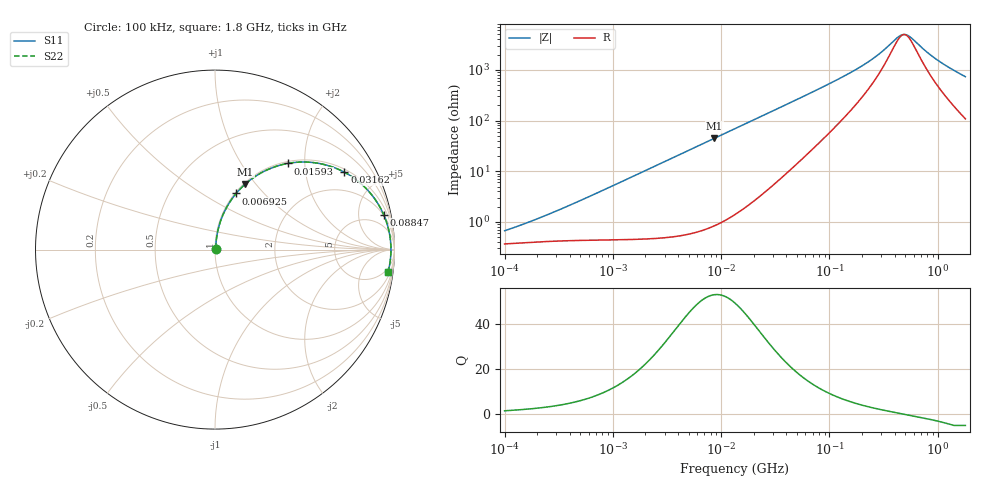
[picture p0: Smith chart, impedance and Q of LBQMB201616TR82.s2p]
! LBQMB201616TR82  S-PARAMETER MODEL  ( General Type )
! Model Generated by TAIYO YUDEN Corporation (http://www.ty-top.com)
! Version 1.0
! TAIYO YUDEN Control No. 191025NI43SB-FBB
! Copyright(c) 2019 TAIYO YUDEN CO.,LTD. All Rights Reserved.
! Product Description (link to TY-COMPAS)
! https://ds.yuden.co.jp/TYCOMPAS/or/detail?pn=LBQMB201616TR82J&u=M
! Products Name : Inductors
! Characteristics :
!  Inductance : 0.82 uH , SRF(min) : 250 MHz , DC Resistance(max) : 0.442 Ohm , Rated Current : 390 mA
!  Case Size : 2.0 x 1.6 / 0.079 x 0.063 [mm/inch] , Thickness : 1.6 / 0.063 [mm/inch]
!  (Conditions: Temperature = 25 degC , DC Bias Current/Voltage = 0A / 0V)
! External Node Assignments :
!  1  o---GGG---o  2
! GND o---------o GND
! Frequency Range : 0.1MHz  -  1800MHz  [ 402 STEP ]
# MHz S RI R 50
! Freq[MHz].  S11 Real  S11 Imag  S21 Real  S21 Imag  S12 Real  S12 Imag  S22 Real  S22 Imag
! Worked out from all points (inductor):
!   401 points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, 100 kHz to 1.8 GHz, reference 50 ohm
!   read as one part in series: L = 844 nH near 230 kHz
!   highest Q = 53.2 at 8.633 MHz (marker M1), where L = 820 nH
!   self-resonance near 489.8 MHz
!   S11 on the Smith chart (normalised r, x): 100 kHz: 1.01, +0.01; 6.925 MHz: 1.01, +0.71; 15.93 MHz: 1.04, +1.64; 31.62 MHz: 1.12, +3.27; 88.47 MHz: 1.89, +9.34; 1.8 GHz: 3, -15
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0.1  0.0037 0.00556  0.9963 -0.00556  0.9963 -0.00556  0.0037 0.00556
0.203473  0.00413 0.0109  0.9959 -0.0109  0.9959 -0.0109  0.00413 0.0109
0.516129  0.00502 0.0266  0.995 -0.0266  0.995 -0.0266  0.00502 0.0266
1.309209  0.00894 0.0667  0.9911 -0.0667  0.9911 -0.0667  0.00894 0.0667
2.66389  0.023 0.1335  0.977 -0.1335  0.977 -0.1335  0.023 0.1335
4.566214  0.0571 0.2206  0.9429 -0.2206  0.9429 -0.2206  0.0571 0.2206
6.92477  0.1177 0.3127  0.8823 -0.3127  0.8823 -0.3127  0.1177 0.3127
8.632747  0.1699 0.3662  0.8301 -0.3662  0.8301 -0.3662  0.1699 0.3662
13.41641  0.3269 0.4591  0.6731 -0.4591  0.6731 -0.4591  0.3269 0.4591
15.92588  0.4049 0.4801  0.5951 -0.4801  0.5951 -0.4801  0.4049 0.4801
21.89777  0.5594 0.4834  0.4406 -0.4834  0.4406 -0.4834  0.5594 0.4834
31.62078  0.7208 0.4312  0.2792 -0.4312  0.2792 -0.4312  0.7208 0.4312
45.66099  0.837 0.3455  0.163 -0.3455  0.163 -0.3455  0.837 0.3455
69.24595  0.9138 0.246  0.0862 -0.246  0.0862 -0.246  0.9138 0.246
88.46596  0.9395 0.1954  0.0605 -0.1954  0.0605 -0.1954  0.9395 0.1954
208.5031  0.9749 0.0728  0.0251 -0.0728  0.0251 -0.0728  0.9749 0.0728
279.7504  0.9783 0.0448  0.0217 -0.0448  0.0217 -0.0448  0.9783 0.0448
357.3983  0.9798 0.0244  0.0202 -0.0244  0.0202 -0.0244  0.9798 0.0244
445.5497  0.9803 0.00722  0.0197 -0.00722  0.0197 -0.00722  0.9803 0.00722
516.0898  0.9804 -0.00399  0.0196 0.00399  0.0196 0.00399  0.9804 -0.00399
975.7037  0.9771 -0.0566  0.0229 0.0566  0.0229 0.0566  0.9771 -0.0566
1800  0.9635 -0.1274  0.0365 0.1274  0.0365 0.1274  0.9635 -0.1274
